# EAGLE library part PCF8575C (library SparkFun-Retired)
PCF8575C I/O Expander. RETIRED IC-08153 (Also move to special)
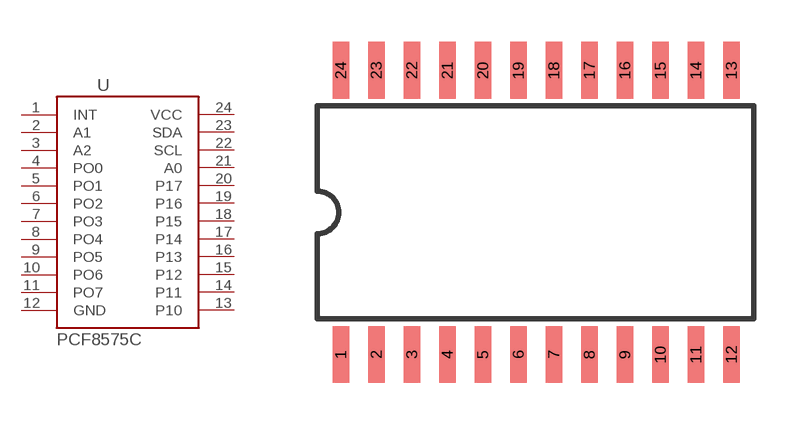
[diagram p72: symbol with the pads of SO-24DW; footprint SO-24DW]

Designator prefix -

## PCF8575C  [SO-24DW]
1  INT
2  A1
3  A2
4  PO0
5  PO1
6  PO2
7  PO3
8  PO4
9  PO5
10  PO6
11  PO7
12  GND
13  P10
14  P11
15  P12
16  P13
17  P14
18  P15
19  P16
20  P17
21  A0
22  SCL
23  SDA
24  VCC

## Footprint SO-24DW (pad centres in mm)
300-mil body, package type SO
smd 0.584 x 2.032: 1 -6.35,-5.08; 2 -5.08,-5.08; 3 -3.81,-5.08; 4 -2.54,-5.08; 5 -1.27,-5.08; 6 0,-5.08; 7 1.27,-5.08; 8 2.54,-5.08; 9 3.81,-5.08; 10 5.08,-5.08; 11 6.35,-5.08; 12 7.62,-5.08; 13 7.62,5.08; 14 6.35,5.08; 15 5.08,5.08; 16 3.81,5.08; 17 2.54,5.08; 18 1.27,5.08; 19 0,5.08; 20 -1.27,5.08; 21 -2.54,5.08; 22 -3.81,5.08; 23 -5.08,5.08; 24 -6.35,5.08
